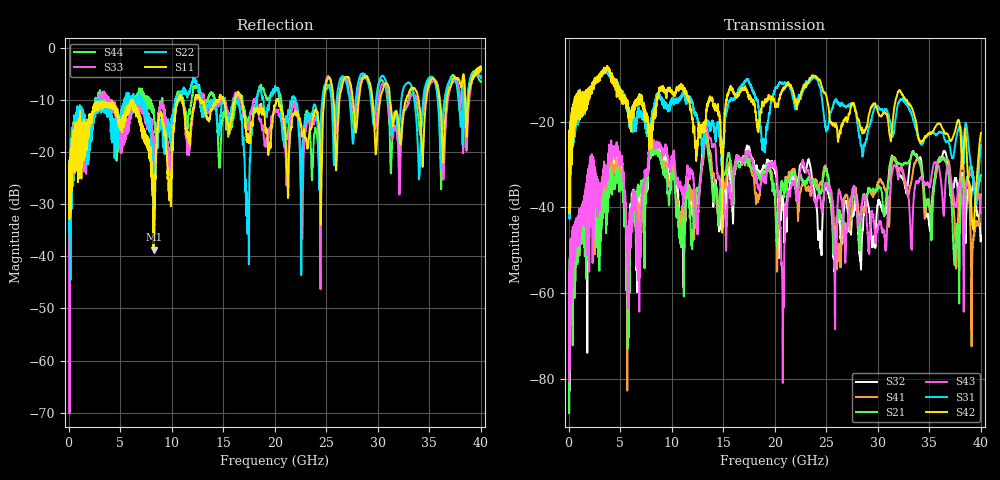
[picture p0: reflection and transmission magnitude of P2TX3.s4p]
!Agilent Technologies,N5245A,MY49151084,A.09.20.08
!Agilent N5245A: A.09.20.08
!Date: Thursday, March 01, 2012 14:04:44
!Correction: S11(Full 4 Port(1,2,3,4))
!S12(Full 4 Port(1,2,3,4))
!S13(Full 4 Port(1,2,3,4))
!S14(Full 4 Port(1,2,3,4))
!S21(Full 4 Port(1,2,3,4))
!S22(Full 4 Port(1,2,3,4))
!S23(Full 4 Port(1,2,3,4))
!S24(Full 4 Port(1,2,3,4))
!S31(Full 4 Port(1,2,3,4))
!S32(Full 4 Port(1,2,3,4))
!S33(Full 4 Port(1,2,3,4))
!S34(Full 4 Port(1,2,3,4))
!S41(Full 4 Port(1,2,3,4))
!S42(Full 4 Port(1,2,3,4))
!S43(Full 4 Port(1,2,3,4))
!S44(Full 4 Port(1,2,3,4))
!S4P File: Measurements: <S11,S12,S13,S14>,
!<S21,S22,S23,S24>,
!<S31,S32,S33,S34>,
!<S41,S42,S43,S44>:
# Hz S  dB  R 50
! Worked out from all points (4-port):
!   3996 points, 50 MHz to 40 GHz, reference 50 ohm
!   strongest paths, dB at 50 MHz, 10.04 GHz, 20.03 GHz, 30.02 GHz, 40 GHz:
!     S42: -26.6, -13.0, -16.4, -17.8, -22.7
!     S31: -25.5, -15.3, -12.3, -16.5, -25.5
!     S43: -59.9, -28.8, -29.3, -44.5, -41.3
!     S21: -57.9, -32.1, -37.8, -34.9, -32.5
!     S41: -57.2, -31.5, -36.3, -34.3, -37.0
!     S32: -65.2, -29.6, -31.1, -39.0, -47.1
!   lowest |S11| = -38.7 dB at 8.28 GHz (marker M1), VSWR 1.02, Z = 48.9 + j0.442 ohm
!   |S11| at or under -10 dB: start of sweep to 6.099 GHz; 6.222 GHz to 10.56 GHz (4.338 GHz wide, 51.7 % of centre); 20.35 GHz to 24.78 GHz (4.429 GHz wide, 19.6 % of centre)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
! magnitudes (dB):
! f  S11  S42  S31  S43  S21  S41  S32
! 50 MHz  -24.1  -26.6  -25.5  -59.9  -57.9  -57.2  -65.2
! 5.79 GHz  -11.3  -17.5  -17.6  -51.2  -60.4  -63.9  -48.4
! 8.28 GHz  -38.7  -18.2  -16.4  -24.6  -26.3  -25.8  -25.7
! 19.88 GHz  -12.2  -14.6  -13.5  -30.6  -34.4  -36.0  -30.0
! 20.76 GHz  -12.6  -12.4  -10.9  -65.5  -34.4  -34.8  -37.7
! 22.71 GHz  -16.9  -12.2  -13.0  -28.9  -33.7  -34.3  -30.3
! 40 GHz  -4.1  -22.7  -25.5  -41.3  -32.5  -37.0  -47.1
